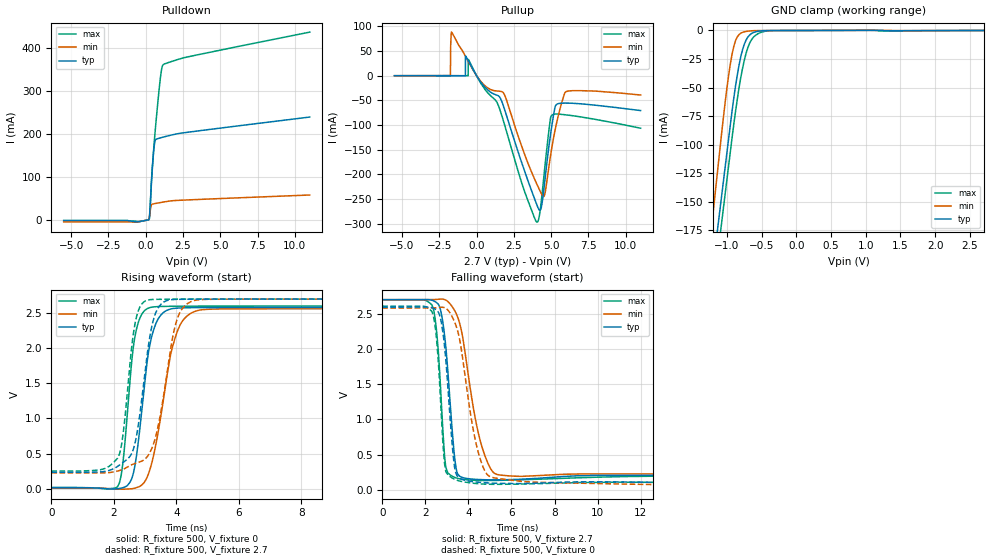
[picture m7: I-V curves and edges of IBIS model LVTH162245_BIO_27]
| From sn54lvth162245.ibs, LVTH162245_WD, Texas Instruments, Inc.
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[Model]   LVTH162245_BIO_27
Model_type  I/O
Vinl = 0.8
Vinh = 2.0
Enable   Active-Low
Vref =   0
Rref =   500
Cref =   50p
Vmeas =   1.5
| variable   typ   min   max
C_comp   10.0pF   NA   NA
| C_pullup   6.88pF   2.16pF   12.65pF
| C_pulldown   5.60pF   4.68pF   7.02pF
| C_tri-state   5.54pF   4.53pF   7.14pF
[Temperature Range]   40   -40   100
| Ambient temperature   25   -40   85
[Voltage range]   2.7   2.7   2.7
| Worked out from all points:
|   slope of the pulldown table from 0 to 0.405 V, typ, clamps not added: 4.09 ohm
|   slope of the pullup table from 0 to 0.405 V, typ, clamps not added: 22.8 ohm
|   GND clamp passes 1 mA (typ) near -0.57 V on its own axis
|   rising waveform, R_fixture 500, V_fixture 0: 20-80 % time 420ps typ, 604ps min, 317ps max; typ from 0.013 V to 2.58 V
|   falling waveform, R_fixture 500, V_fixture 2.7: 20-80 % time 393ps typ, 819ps min, 302ps max; typ from 2.7 V to 0.226 V
|   rising waveform, R_fixture 500, V_fixture 2.7: 20-80 % time 454ps typ, 579ps min, 343ps max; typ from 0.234 V to 2.7 V
|   falling waveform, R_fixture 500, V_fixture 0: 20-80 % time 403ps typ, 833ps min, 313ps max; typ from 2.59 V to 0.015 V
[GND Clamp]
| LVTH162245_BIO_27
|   Voltage   I(typ)   I(min)   I(max)
-5.5V     -2.928A    -3.105A    -2.935A
-1.26V    -236.7mA   -194.1mA   -261.3mA
-1.185V   -199.1mA   -151.5mA   -222.8mA
-1.075V   -144.2mA   -89.15mA   -167.7mA
-975mV    -94.48mA   -38.99mA   -118.1mA
-875mV    -48.18mA   -8.698mA   -70.33mA
-800mV    -22.74mA   -2.357mA   -40.93mA
-750mV    -12.09mA   -1.161mA   -26.11mA
-675mV    -4.043mA   -444.8uA   -11.37mA
-600mV    -1.388mA   -150.7uA   -4.764mA
-325mV    -65.11uA   -60.21uA   -90.18uA
2.7V      25.89pA    18.52pA    1.804nA
[Pulldown]
| LVTH162245_BIO_27
|   Voltage   I(typ)   I(min)   I(max)
-5.5V     -189uA     -3.419mA   -1.741mA
-635mV    -3.429mA   -4.205mA   -2.236mA
225mV     3.425mA    4.813mA    2.084mA
285mV     28.13mA    17.72mA    17.13mA
375mV     81.45mA    35.06mA    86.58mA
500mV     146.9mA    37.96mA    150mA
600mV     179.4mA    38.65mA    193.1mA
685mV     187.4mA    39.23mA    226.4mA
990mV     190.9mA    41.22mA    331.6mA
1.09V     191.9mA    41.84mA    353.7mA
1.19V     192.8mA    42.44mA    360.7mA
11V       239.1mA    58.62mA    435.7mA
[Pullup]
| LVTH162245_BIO_27
|   Voltage   I(typ)   I(min)   I(max)
-5.5V     57.02uA    34.21uA    92.9uA
-1.76V    50.14uA    300.4uA    80.13uA
-1.735V   50.09uA    60.63mA    80.04uA
-1.685V   49.98uA    88.55mA    79.84uA
-565mV    31.04mA    29.25mA    55.03uA
-540mV    29.62mA    27.87mA    32.84mA
1.84V     -64.86mA   -36.42mA   -95.58mA
4.05V     -262.4mA   -220.4mA   -297.1mA
4.54V     -223.4mA   -243.7mA   -196.6mA
5.045V    -102mA     -146.3mA   -80.03mA
5.99V     -55.5mA    -32.44mA   -79.42mA
11V       -70.65mA   -39.08mA   -106.4mA
[Ramp]
| LVTH162245_BIO_27
| variable   typ   min   max
dV/dt_r   1.55/4.27E-10   1.54/6.13E-10   1.56/3.23E-10
dV/dt_f   1.54/4.08E-10   1.51/8.44E-10   1.54/3.17E-10
R_load = 500
[Rising Waveform]
| LVTH162245_BIO_27
R_fixture =   500
C_fixture =   0
L_fixture =   0
V_fixture =   0
V_fixture_min = 0
V_fixture_max = 0
|   Time   V(typ)   V(min)   V(max)
0s        12.83mV    8.193mV    16.39mV
2.135ns   -800.2uV   -6.121mV   39.39mV
2.295ns   13.83mV    -7.81mV    387.5mV
2.57ns    140.3mV    -1.996mV   1.798V
2.695ns   380.9mV    9.545mV    2.209V
3.075ns   1.835V     172.2mV    2.564V
3.275ns   2.26V      476.9mV    2.588V
4.005ns   2.57V      2.205V     2.598V
4.865ns   2.579V     2.55V      2.599V
50ns      2.582V     2.563V     2.601V
[Falling Waveform]
| LVTH162245_BIO_27
R_fixture =   500
C_fixture =   0
L_fixture =   0
V_fixture =   2.7
V_fixture_min = 2.7
V_fixture_max = 2.7
|   Time   V(typ)   V(min)   V(max)
0s        2.7V       2.7V       2.7V
2.305ns   2.693V     2.702V     2.626V
2.475ns   2.668V     2.703V     2.386V
2.64ns    2.615V     2.707V     1.803V
2.955ns   2.022V     2.694V     327.8mV
3.365ns   452.2mV    2.544V     177.4mV
3.66ns    185mV      2.285V     153.5mV
4.55ns    146.5mV    698.9mV    133.7mV
5.46ns    143.6mV    211.1mV    135.6mV
50ns      225.7mV    225.6mV    240.8mV
[Rising Waveform]
| LVTH162245_BIO_27
R_fixture =   500
C_fixture =   0
L_fixture =   0
V_fixture =   2.7
V_fixture_min = 2.7
V_fixture_max = 2.7
|   Time   V(typ)   V(min)   V(max)
0s        233.6mV    225.6mV    250.7mV
2.115ns   315.1mV    249.7mV    430.7mV
2.29ns    371.2mV    274.3mV    758.9mV
2.565ns   495.7mV    338.6mV    1.989V
2.69ns    669.7mV    359.1mV    2.375V
3.155ns   2.168V     516.8mV    2.691V
3.445ns   2.591V     948.4mV    2.696V
4.015ns   2.695V     2.396V     2.699V
4.71ns    2.699V     2.69V      2.7V
50ns      2.7V       2.7V       2.7V
[Falling Waveform]
| LVTH162245_BIO_27
R_fixture =   500
C_fixture =   0
L_fixture =   0
V_fixture =   0
V_fixture_min = 0
V_fixture_max = 0
|   Time   V(typ)   V(min)   V(max)
0s        2.594V     2.582V     2.608V
2.275ns   2.59V      2.583V     2.542V
2.62ns    2.515V     2.589V     1.746V
2.945ns   1.87V      2.579V     273.8mV
3.355ns   329.8mV    2.388V     151.6mV
3.82ns    137.5mV    1.679V     111.9mV
4.285ns   114.4mV    762.6mV    92.57mV
4.745ns   102.2mV    280.8mV    82.41mV
6.285ns   89.54mV    126.3mV    81.61mV
50ns      15.39mV    10.32mV    19.95mV
